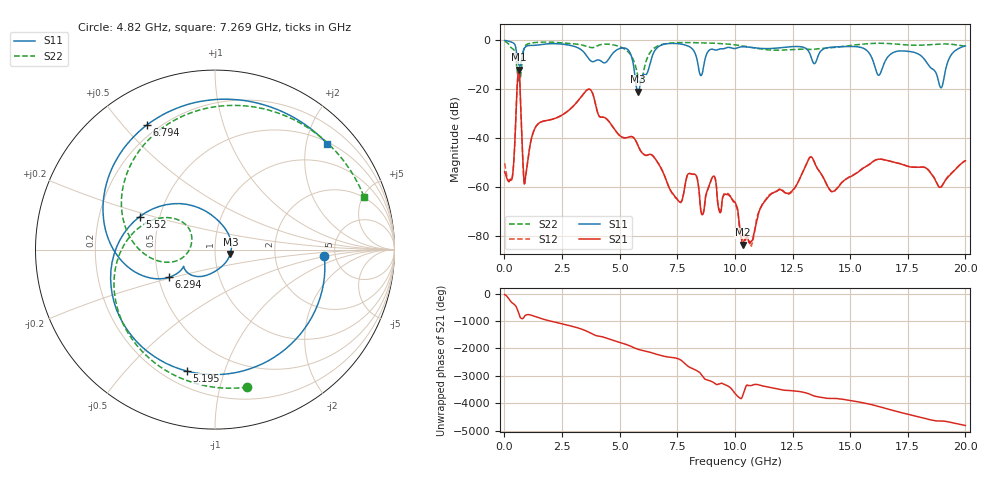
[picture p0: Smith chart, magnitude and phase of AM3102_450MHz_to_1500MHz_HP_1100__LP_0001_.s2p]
!Agilent Technologies,E8364B,MY43040894,A.07.50.67
!Agilent E8364B: A.07.50.67
!Date: Thursday, January 11, 2018 06:32:02
!Correction: S11(Full 2 Port(1,2))
!S21(Full 2 Port(1,2))
!S12(Full 2 Port(1,2))
!S22(Full 2 Port(1,2))
!S2P File: Measurements: S11, S21, S12, S22:
# Hz S  dB  R 50
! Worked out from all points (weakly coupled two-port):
!   1601 points, 10 MHz to 20 GHz, reference 50 ohm
!   highest |S21| = -11.97 dB at 622.2 MHz (marker M1); lowest = -83.4 dB at 10.34 GHz (marker M2)
!   lowest |S11| = -21.0 dB at 5.795 GHz (marker M3), VSWR 1.19, Z = 59.3 - j2.91 ohm
!   |S11| at or under -10 dB: 5.597 GHz to 6.307 GHz (709.4 MHz wide, 11.9 % of centre); 16.05 GHz to 16.45 GHz (399.9 MHz wide, 2.46 % of centre); 18.38 GHz to 19.2 GHz (811.3 MHz wide, 4.32 % of centre)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
!   |S22| runs from -17.4 to -0.4 dB; largest |S21 - S12| = 0.031
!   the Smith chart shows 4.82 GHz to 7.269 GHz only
!   S11 on the Smith chart (normalised r, x): 4.82 GHz: 4.07, -0.48; 5.195 GHz: 0.29, -0.75; 5.52 GHz: 0.38, +0.18; 6.294 GHz: 0.57, -0.19; 6.794 GHz: 0.16, +0.58; 7.269 GHz: 0.53, +2.42
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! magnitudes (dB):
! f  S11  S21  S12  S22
! 10 MHz  -0.1  -53.6  -50.1  -0.4
! 322.3 MHz  -0.8  -56.7  -56.9  -3.2
! 622.2 MHz  -9.9  -12.0  -12.0  -16.4
! 909.5 MHz  -2.8  -56.3  -56.4  -2.2
! 1.397 GHz  -2.0  -34.8  -34.8  -0.9
! 3.346 GHz  -4.0  -22.9  -22.9  -1.9
! 4.82 GHz  -4.3  -36.9  -36.9  -2.1
! 5.195 GHz  -3.2  -39.8  -39.8  -3.5
! 5.52 GHz  -6.8  -39.3  -39.3  -6.6
! 5.795 GHz  -21.0  -42.9  -42.9  -14.9
! 6.294 GHz  -10.4  -46.6  -46.6  -5.4
! 6.682 GHz  -2.6  -50.3  -50.2  -2.2
! 6.794 GHz  -2.0  -52.2  -52.0  -1.8
! 7.269 GHz  -1.3  -62.2  -62.3  -1.1
! 8.531 GHz  -14.4  -69.9  -69.7  -1.0
! 10.01 GHz  -3.4  -66.1  -66.5  -1.9
! 10.34 GHz  -2.7  -83.4  -81.1  -2.3
! 13.34 GHz  -7.8  -47.8  -47.8  -3.8
! 14.24 GHz  -2.8  -61.7  -61.8  -3.0
! 16.68 GHz  -6.4  -49.2  -49.2  -1.3
! 18.94 GHz  -19.4  -59.9  -59.9  -1.5
! 20 GHz  -2.3  -49.2  -49.1  -2.4
